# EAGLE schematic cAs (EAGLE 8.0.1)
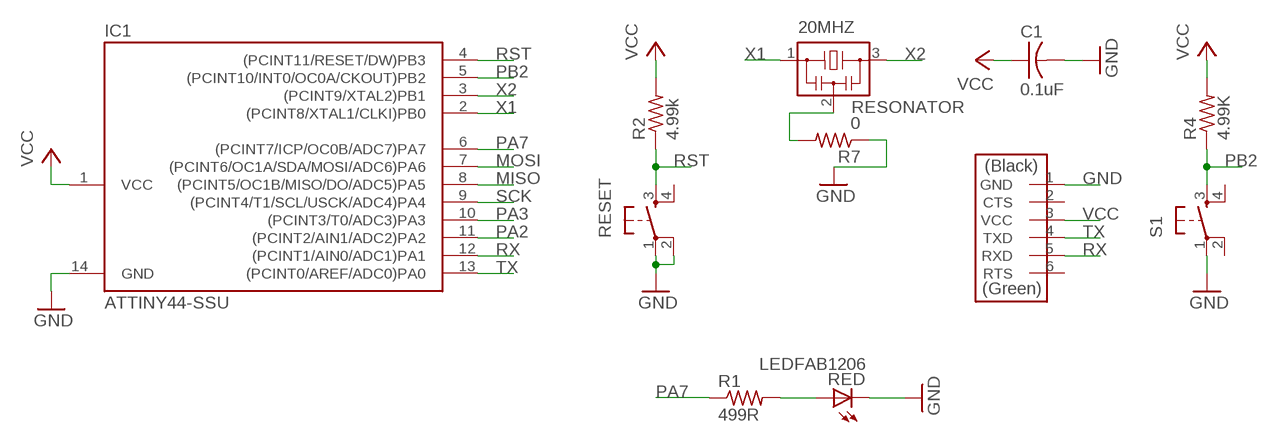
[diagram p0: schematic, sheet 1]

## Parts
20MHZ  RESONATOR  [EFOBM]
C1  0.1uF  CAP-US1206K  [C1206K]
FTDI  FTDI-SMD-HEADER  [1X06SMD]
IC1  ATTINY44-SSU  [SOIC14]
R1  499R  RES-US1206FAB  [R1206FAB]
R2  4.99k  RES-US1206FAB  [R1206FAB]
R4  4.99K  RES-US1206FAB  [R1206FAB]
R7  0  RES-US1206FAB  [R1206FAB]
RED  LEDFAB1206  [LED1206FAB]
RESET  6MM_SWITCH6MM_SWITCH  [6MM_SWITCH]
S1  6MM_SWITCH6MM_SWITCH  [6MM_SWITCH]

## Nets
GND: C1.2 FTDI.1(GND) IC1.14(GND) R7.1 RED.2(C) RESET.1(P) RESET.2(P1) S1.1(P)
MISO: IC1.8((PCINT5/OC1B/MISO/DO/ADC5)PA5)
MOSI: IC1.7((PCINT6/OC1A/SDA/MOSI/ADC6)PA6)
N$1: R1.2 RED.1(A)
N$2: 20MHZ.2 R7.2
PA2: IC1.11((PCINT2/AIN1/ADC2)PA2)
PA3: IC1.10((PCINT3/T0/ADC3)PA3)
PA7: IC1.6((PCINT7/ICP/OC0B/ADC7)PA7) R1.1
PB2: IC1.5((PCINT10/INT0/OC0A/CKOUT)PB2) R4.1 S1.3(S)
RST: IC1.4((PCINT11/RESET/DW)PB3) R2.1 RESET.3(S)
RX: FTDI.5(RXD) IC1.12((PCINT1/AIN0/ADC1)PA1)
SCK: IC1.9((PCINT4/T1/SCL/USCK/ADC4)PA4)
TX: FTDI.4(TXD) IC1.13((PCINT0/AREF/ADC0)PA0)
VCC: C1.1 FTDI.3(VCC) IC1.1(VCC) R2.2 R4.2
X1: 20MHZ.1 IC1.2((PCINT8/XTAL1/CLKI)PB0)
X2: 20MHZ.3 IC1.3((PCINT9/XTAL2)PB1)
Unconnected: FTDI.2(CTS) FTDI.6(RTS) RESET.4(S1) S1.2(P1) S1.4(S1)

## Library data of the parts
20MHZ = fab:RESONATOR
C1 = fab:CAP-US
FTDI = fab:FTDI-SMD-HEADER
IC1 = fab:ATTINY44
R1 R2 R4 R7 = fab:RES-US: Resistor (US Symbol)
RED = fab:LED: LED
RESET S1 = fab:6MM_SWITCH: OMRON SWITCH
